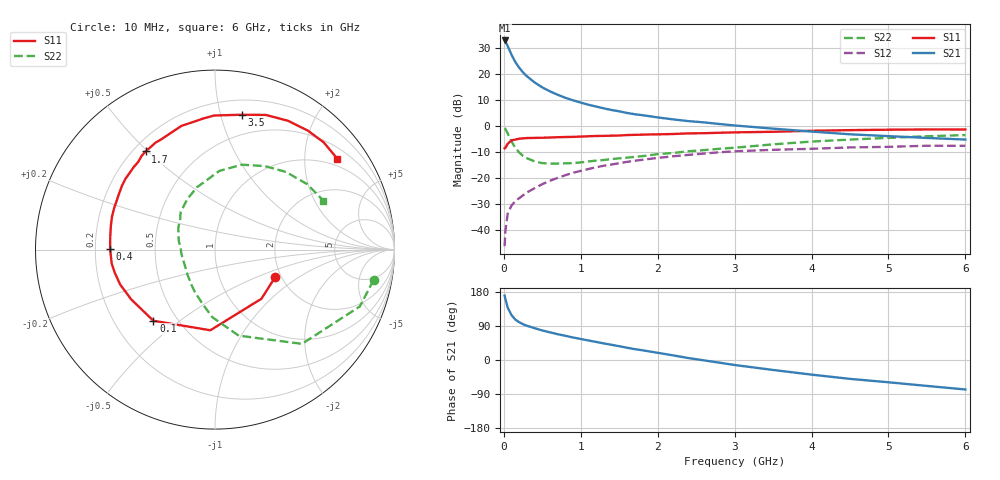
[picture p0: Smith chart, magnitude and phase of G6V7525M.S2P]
! SIEMENS Small Signal Semiconductors
! BFG193
! Si NPN RF Bipolar Junction Transistor in SOT223
! VCE = 0.75 V  IC = 25 mA
! Common Emitter S-Parameters:  August  1996
# GHz  S  MA  R  50
!  f  S11  S21  S12  S22
! GHz  MAG  ANG  MAG  ANG  MAG  ANG  MAG  ANG
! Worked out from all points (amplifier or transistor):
!   36 points, 10 MHz to 6 GHz, reference 50 ohm
!   highest |S21| = 32.9 dB at 10 MHz (marker M1)
!   |S21| within 3 dB of that: start of sweep to 62.63 MHz
!   unconditionally stable (mu >= 1): 466 MHz to 4.041 GHz
!   at 250 MHz: K = 0.83, MSG = 23.7 dB, |S12| = -26.7 dB
!   at 1.4 GHz: K = 1.08, MAG = 8.8 dB, |S12| = -14.9 dB
!   at 6 GHz: K = 0.99, MSG = 1.2 dB, |S12| = -7.7 dB
!   S11 on the Smith chart (normalised r, x): 10 MHz: 1.86, -0.66; 100 MHz: 0.37, -0.40; 400 MHz: 0.26, +0.00; 1.7 GHz: 0.25, +0.49; 3.5 GHz: 0.32, +1.17; 6 GHz: 0.78, +2.83
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0.01  0.3685 -24.6  44.05 169.9  0.0048 82.4  0.8997 -10.8
0.02  0.3768 -46.6  42.25 161.3  0.0094 76.4  0.8672 -21.4
0.05  0.4501 -93.3  34.36 138.5  0.0203 61.7  0.7146 -47.3
0.1  0.5243 -130.9  23.41 118.3  0.0292 54.5  0.4973 -74.6
0.15  0.5431 -149.3  16.83 106.5  0.0354 51.8  0.3763 -92.4
0.2  0.5633 -159.9  13.14 99.6  0.0404 53.4  0.3059 -103.8
0.25  0.5731 -167.0  10.67 94.4  0.046 54.6  0.2621 -115.2
0.3  0.5808 -172.4  9.003 90.3  0.0519 56.1  0.2371 -123.4
0.4  0.5845 179.5  6.839 84.0  0.0628 57.6  0.206 -138.6
0.5  0.5884 172.6  5.491 78.0  0.0752 57.5  0.1912 -150.4
0.6  0.5947 167.4  4.598 73.0  0.0874 57.3  0.187 -159.5
0.7  0.6026 162.2  3.962 68.1  0.0993 56.3  0.1872 -167.8
0.9  0.612 153.4  3.097 59.4  0.1245 53.2  0.1911 177.8
1.1  0.6285 145.5  2.545 51.5  0.1471 49.9  0.2061 167.5
1.4  0.6453 134.7  2.015 40.1  0.1796 43.2  0.2284 153.2
1.7  0.6699 125.3  1.672 28.7  0.2117 36.7  0.2513 141.2
2.2  0.6953 110.6  1.329 12.2  0.2588 24.3  0.2996 125.3
2.8  0.734 94.9  1.084 -7.0  0.309 9.7  0.361 106.5
3.5  0.7667 78.6  0.881 -26.3  0.3446 -8.0  0.4393 86.8
4.5  0.8249 60.5  0.686 -49.8  0.3831 -27.1  0.5424 59.0
5.5  0.8507 44.6  0.584 -68.4  0.4128 -49.1  0.6292 35.5
6  0.849 36.6  0.543 -77.8  0.4115 -61.5  0.663 24.3
